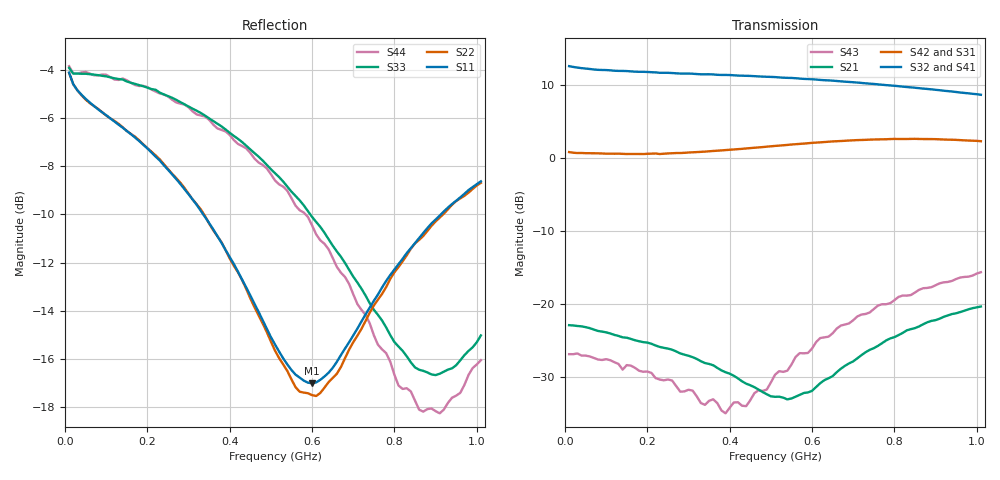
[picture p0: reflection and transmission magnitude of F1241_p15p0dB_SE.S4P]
! Integrated Device Technology
! Corporate Headquarters
! 6024 Silver Creek Valley Road
! San Jose, CA 95138  USA
! Phone:  1-408-284-8200
! Toll Free:  1-800-223-1366
! Webpage:  http://www.idt.com/
! Timing and RF Division
! 515 Groton Road, Suite 102
! Westford, MA 01886-6024
! Device:  F1241
! Description: Dual Intermediate Frequency Digital Variable Gain Amplifier
! Frequency:  10.0 -  500.00 MHz
! Package:  5x5 mm QFN Plastic Package: 32 pin
! Ports:  8 RF, 20 DC
!  Pin  1  = GA3  Pin 17  = RF OUT_B+
!  Pin  2  = GA4  Pin 18  = RF OUT_B-
!  Pin  3  = GA5  Pin 19  = STBY_B
!  Pin  4  = ISET_A  Pin 20  = Ground
!  Pin  5  = ISET_B  Pin 21  = Ground
!  Pin  6  = GB5  Pin 22  = STB_A
!  Pin  7  = GB4  Pin 23  = RF OUT_A-  = Port 4
!  Pin  8  = GB3  Pin 24  = RF OUT_A+  = Port 3
!  Pin  9  = GB2  Pin 25  = NO CONNECT
!  Pin 10  = GB1  Pin 26  = NO CONNECT
!  Pin 11  = RF IN_B+  Pin 27  = VCC
!  Pin 12  = RF IN_B-  Pin 28  = Ground
!  Pin 13  = Ground  Pin 29  = RF IN_A-  = Port 2
!  Pin 14  = VCC  Pin 30  = RF IN_A+  = Port 1
!  Pin 15  = NO CONNECT  Pin 31  = GA1
!  Pin 16  = NO CONNECT  Pin 32  = GA2
! State:  5
! Gain State:  15.0 dB
! Voltages:  Vcc = +5.00 Volts  Icc approximately 160.0 mA or 80 mA per channel.
! Data:  The device was measured on a custom evaluation board which has
!  individual transmission lines to the RF pins.  Data was collected
!  using a calibrated network analyzer.  The evaluation board was
!  de-embedded using a port reference technique.
!  The reference plane is the edge of the package pin.
!  Only Channel A was measured.
!  This data is in single-ended operation.  If your needs are balanced
!  or differential S-parameters then this file needs to be used a
!  linear simulator.
! Misc:  Lot Code  160028MY
!  Action Tracker AT004
! Date Measured:  2014-08-14
! Date:  2014-08-28  MJV
! Note:
!  Integrated Device Technology supplies this data as a sample of measured
!  data at the package pin for this product.  Your particular data for this
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# Hz S dB R 50
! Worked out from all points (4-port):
!   101 points, 10 MHz to 1.01 GHz, reference 50 ohm
!   strongest paths, dB at 10 MHz, 260 MHz, 510 MHz, 760 MHz, 1.01 GHz:
!     S32: 12.5, 11.6, 11.1, 10.1, 8.6
!     S41: 12.6, 11.5, 10.9, 9.9, 8.4
!     S42: 0.8, 0.6, 1.6, 2.5, 2.3
!     S31: 0.8, 0.5, 1.3, 2.3, 2.1
!     S21: -22.9, -26.3, -32.7, -25.8, -20.4
!     S43: -26.9, -30.5, -29.7, -20.2, -15.7
!   lowest |S11| = -17.0 dB at 600 MHz (marker M1), VSWR 1.33, Z = 39.4 - j6.81 ohm
!   |S11| at or under -10 dB: 335.6 MHz to 913.1 MHz (577.5 MHz wide, 92.5 % of centre)
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1e7  -4.12 -12.3  -22.93 7.4  -48.65 39.2  -22.10 7.7
     -22.93 7.2  -4.13 -12.2  -22.12 7.4  -48.68 39.3
     0.77 2.9  12.55 -175.8  -3.92 -9.1  -26.96 19.6
     12.57 -175.7  0.78 3.0  -26.90 18.9  -3.85 -9.3
5e7  -5.20 -14.0  -23.26 -10.5  -43.77 53.5  -22.42 -2.8
     -23.20 -10.5  -5.23 -13.6  -22.36 -2.8  -44.03 54.2
     0.64 -4.3  12.22 172.2  -4.16 -5.7  -27.35 -6.2
     12.22 171.9  0.63 -4.2  -27.10 -4.7  -4.08 -5.8
2.5e8  -8.15 -41.1  -26.17 -41.6  -31.91 54.4  -22.56 -9.1
       -26.14 -44.3  -8.11 -39.2  -22.54 -9.5  -31.91 53.9
       0.48 -19.3  11.64 145.8  -5.09 -21.1  -29.65 -55.5
       11.57 145.1  0.59 -19.2  -30.37 -49.2  -5.11 -20.4
3.9e8  -11.48 -65.3  -29.30 -69.0  -28.43 41.7  -22.07 -15.1
       -29.38 -74.9  -11.48 -62.6  -21.97 -14.9  -28.37 40.9
       0.82 -29.0  11.35 128.4  -6.48 -32.9  -30.26 -109.9
       11.25 127.4  1.05 -29.5  -35.00 -111.5  -6.56 -31.3
6e8  -17.02 -143.0  -33.73 -176.1  -25.42 20.9  -21.33 -28.5
     -31.92 178.3  -17.51 -141.8  -21.12 -28.6  -25.32 19.0
     1.77 -47.8  10.76 101.7  -10.10 -55.5  -24.89 167.1
     10.59 100.8  2.04 -49.7  -26.13 149.6  -10.46 -52.7
8.2e8  -11.84 145.6  -25.27 108.1  -23.96 0.2  -21.35 -46.0
       -24.00 109.2  -11.95 145.5  -20.94 -46.3  -23.79 -2.8
       2.35 -74.2  9.75 74.5  -15.67 -100.9  -18.99 119.0
       9.54 73.6  2.57 -77.1  -18.88 102.8  -17.25 -97.7
1.01e9  -8.63 125.1  -21.04 80.8  -23.33 -15.8  -22.01 -60.7
        -20.38 79.8  -8.69 125.5  -21.43 -61.0  -23.17 -19.5
        2.07 -99.4  8.63 52.1  -15.03 -165.5  -16.00 86.0
        8.38 51.4  2.27 -102.8  -15.68 74.8  -16.05 -172.4
